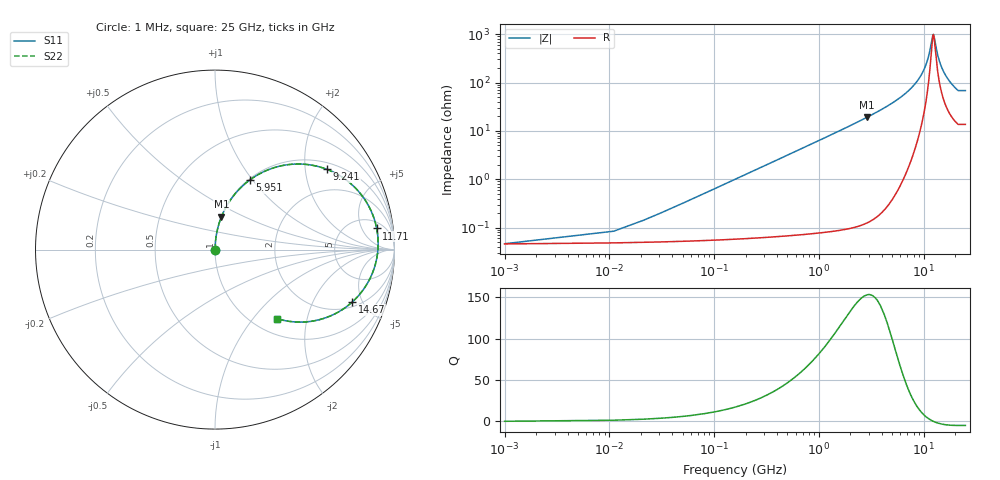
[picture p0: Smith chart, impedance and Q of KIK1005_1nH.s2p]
!version-3
!date-01.2023
!Series
# MHz S RI R 50
!Freq ReS11 ImS11 ReS21 ImS21 ReS12 ImS12 ReS22 ImS22
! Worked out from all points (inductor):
!   2501 points, 1 MHz to 25 GHz, reference 50 ohm
!   read as one part in series: L = 1 nH near 121 MHz
!   highest Q = 153 at 2.871 GHz (marker M1), where L = 1.06 nH
!   self-resonance near 12.38 GHz
!   S11 on the Smith chart (normalised r, x): 1 MHz: 1.00, +0.00; 5.951 GHz: 1.01, +0.97; 9.241 GHz: 1.20, +2.61; 11.71 GHz: 7, +10; 14.67 GHz: 2.35, -4.17; 25 GHz: 1.27, -1.34
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1  0.00046 6.28e-05  0.9995 -6.28e-05  0.9995 -6.28e-05  0.00046 6.28e-05
141  0.000647 0.00885  0.9994 -0.00885  0.9994 -0.00885  0.000647 0.00885
201  0.000751 0.0126  0.9992 -0.0126  0.9992 -0.0126  0.000751 0.0126
351  0.00112 0.022  0.9989 -0.022  0.9989 -0.022  0.00112 0.022
581  0.00203 0.0365  0.998 -0.0365  0.998 -0.0365  0.00203 0.0365
941  0.00428 0.0592  0.9957 -0.0592  0.9957 -0.0592  0.00428 0.0592
1421  0.00895 0.0896  0.9911 -0.0896  0.9911 -0.0896  0.00895 0.0896
2871  0.0362 0.1836  0.9638 -0.1836  0.9638 -0.1836  0.0362 0.1836
4171  0.0822 0.2709  0.9178 -0.2709  0.9178 -0.2709  0.0822 0.2709
5951  0.1952 0.389  0.8048 -0.389  0.8048 -0.389  0.1952 0.389
8341  0.481 0.4765  0.5189 -0.4765  0.5189 -0.4765  0.481 0.4765
9241  0.6231 0.4475  0.3769 -0.4475  0.3769 -0.4475  0.6231 0.4475
10661  0.8239 0.2943  0.1761 -0.2943  0.1761 -0.2943  0.8239 0.2943
11211  0.8742 0.2054  0.1258 -0.2053  0.1258 -0.2053  0.8742 0.2054
11711  0.9009 0.1178  0.0994 -0.1176  0.0994 -0.1176  0.9009 0.1178
12191  0.909 0.033  0.0916 -0.0328  0.0916 -0.0328  0.909 0.033
12501  0.9058 -0.02  0.0943 0.0199  0.0943 0.0199  0.9058 -0.02
13571  0.8545 -0.1785  0.1455 0.1784  0.1455 0.1784  0.8545 -0.1785
14671  0.7654 -0.2913  0.2346 0.2913  0.2346 0.2913  0.7654 -0.2913
16671  0.5953 -0.3867  0.4047 0.3867  0.4047 0.3867  0.5953 -0.3867
20841  0.3625 -0.3893  0.6375 0.3893  0.6375 0.3893  0.3625 -0.3893
25000  0.3458 -0.3844  0.6542 0.3844  0.6542 0.3844  0.3458 -0.3844
